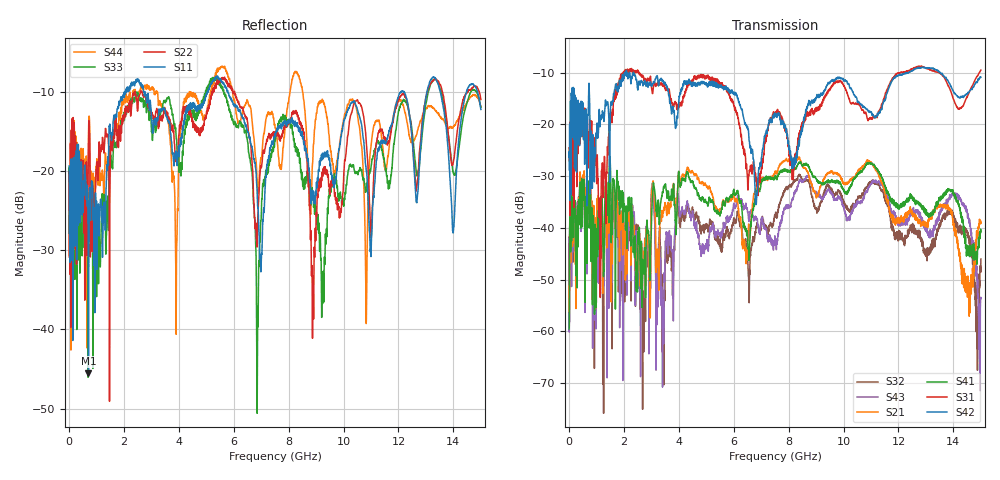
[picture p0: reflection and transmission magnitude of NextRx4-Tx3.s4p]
! FILE: N:\QM 2007\Prüfprotokolle\Highspeed\Konfektionierte Ltg\L45593-D106\D30\8216\0002\Next  Platine 1\NextRx4-Tx3.s4p
# MHz S DB R 50.00
! FREQ  S11  S12  S13  S14
!  S21  S22  S23  S24
!  S31  S32  S33  S34
!  S41  S42  S43  S44
!  DB  ANG  DB  ANG  DB  ANG  DB  ANG
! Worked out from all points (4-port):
!   2999 points, 10 MHz to 15 GHz, reference 50 ohm
!   strongest paths, dB at 10 MHz, 3.755 GHz, 7.505 GHz, 11.26 GHz, 15 GHz:
!     S42: -26.3, -17.0, -18.3, -18.2, -10.9
!     S31: -24.5, -15.8, -18.3, -18.0, -9.5
!     S41: -59.5, -33.7, -30.4, -29.0, -40.9
!     S21: -51.3, -34.0, -29.2, -29.5, -39.0
!     S43: -41.9, -44.2, -42.3, -31.1, -53.7
!     S32: -41.8, -46.7, -37.8, -31.5, -46.0
!   lowest |S11| = -45.5 dB at 715 MHz (marker M1), VSWR 1.01, Z = 49.5 + j0.132 ohm
!   |S11| at or under -10 dB: start of sweep to 2.038 GHz; 2.777 GHz to 5.045 GHz (2.268 GHz wide, 58 % of centre); 5.791 GHz to 12.08 GHz (6.285 GHz wide, 70.4 % of centre)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
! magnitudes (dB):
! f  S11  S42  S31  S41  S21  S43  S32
! 10 MHz  -19.4  -26.3  -24.5  -59.5  -51.3  -41.9  -41.8
! 715 MHz  -45.5  -14.6  -24.1  -33.3  -33.9  -34.2  -34.3
! 3.43 GHz  -12.2  -11.5  -12.3  -33.0  -36.8  -58.1  -60.8
! 6.87 GHz  -24.3  -32.6  -30.8  -32.7  -31.2  -38.9  -39.3
! 7.745 GHz  -14.5  -19.6  -18.4  -28.9  -27.4  -39.0  -34.2
! 14.06 GHz  -23.5  -14.0  -16.0  -34.2  -41.6  -33.5  -39.1
! 15 GHz  -12.2  -10.9  -9.5  -40.9  -39.0  -53.7  -46.0
